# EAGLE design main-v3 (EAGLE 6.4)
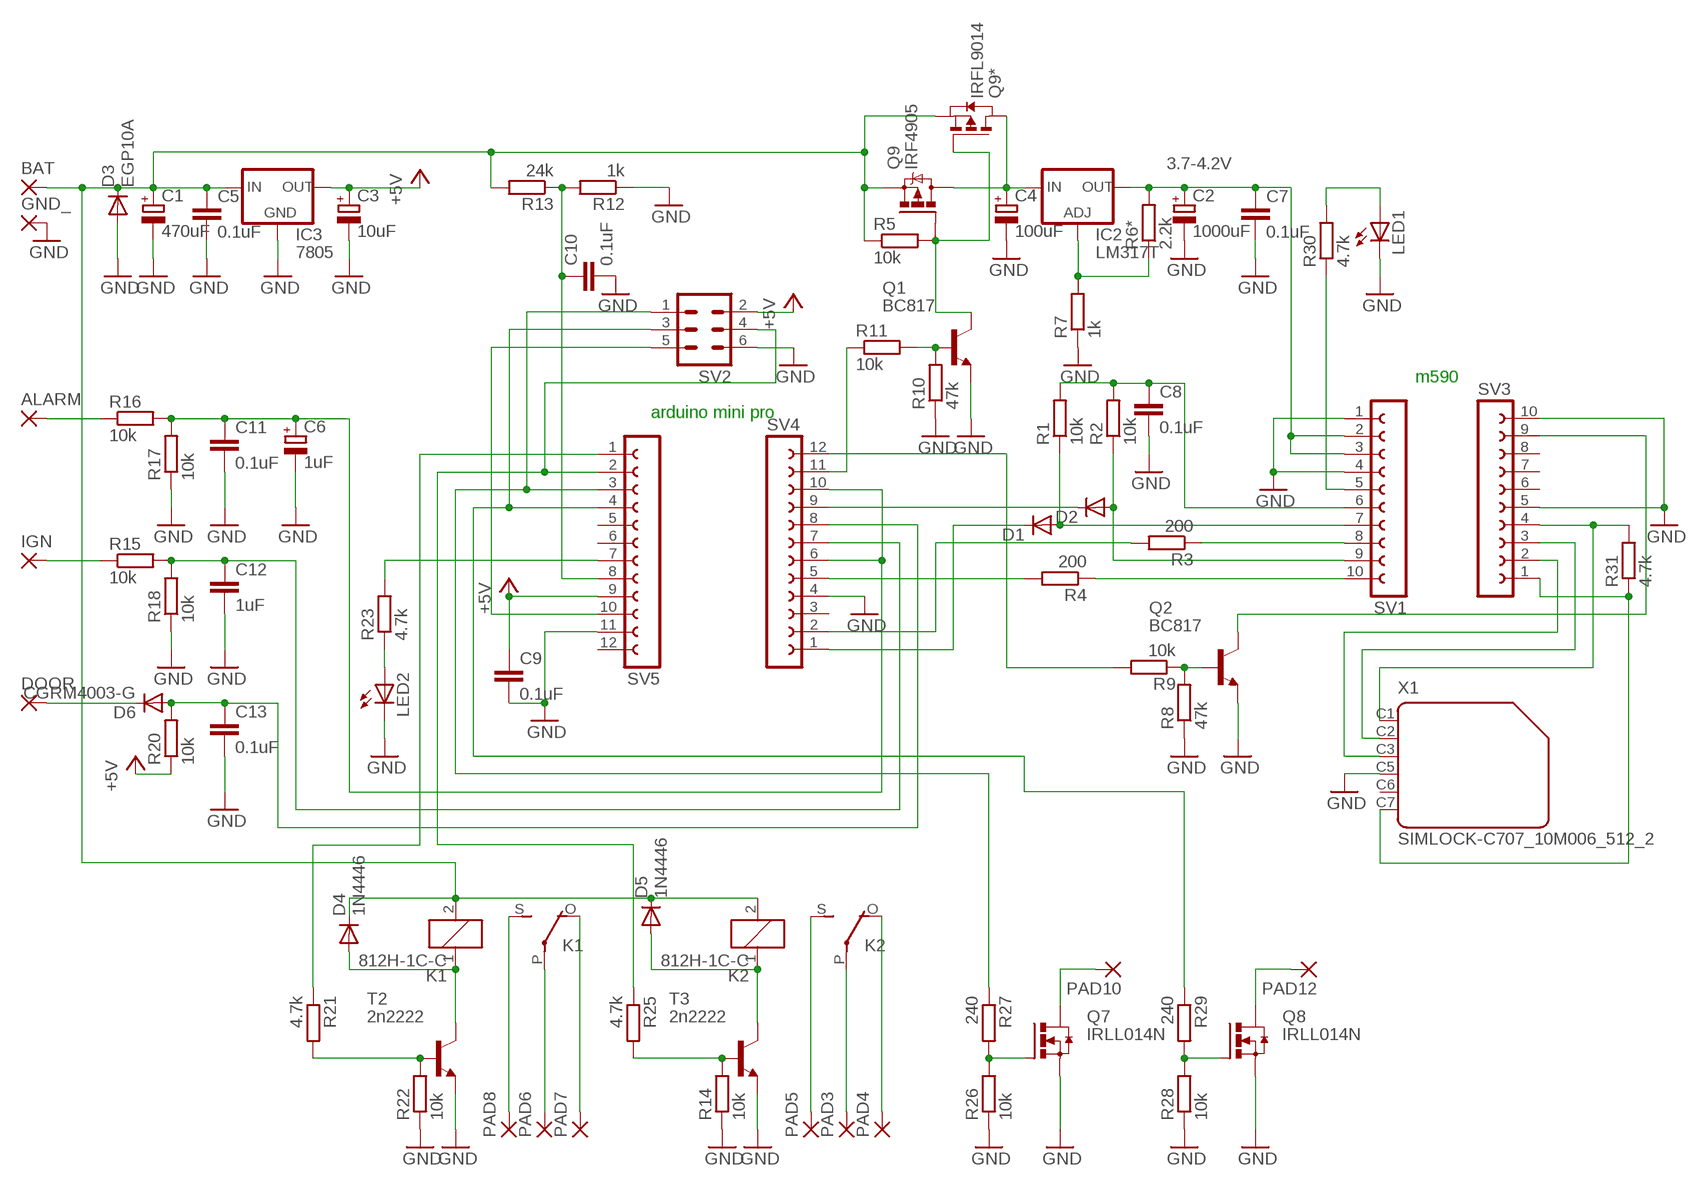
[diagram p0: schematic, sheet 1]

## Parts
ALARM  3,17/1,1  [3,17/1,1]
BAT  3,17/1,1  [3,17/1,1]
C1  470uF  CPOL-EUE5-10.5  [E5-10,5]
C2  1000uF  CPOL-EUE2.5-7  [E2,5-7]
C3  10uF  CPOL-EUE2.5-7  [E2,5-7]
C4  100uF  CPOL-EUE2.5-7  [E2,5-7]
C5  0.1uF  C-EUC1206  [C1206]
C6  1uF  CPOL-EUE2.5-7  [E2,5-7]
C7  0.1uF  C-EUC1206  [C1206]
C8  0.1uF  C-EUC1206  [C1206]
C9  0.1uF  C-EUC1206  [C1206]
C10  0.1uF  C-EUC1206  [C1206]
C11  0.1uF  C-EUC1206  [C1206]
C12  1uF  C-EUC1206  [C1206]
C13  0.1uF  C-EUC1206  [C1206]
D1  BAS15  [DO34-7]
D2  BAS15  [DO34-7]
D3  EGP10A  [DO41-10]
D4  1N4446  [DO35-10]
D5  1N4446  [DO35-10]
D6  CGRM4003-G  [SOD-123_MINI-SMA]
DOOR  3,17/1,1  [3,17/1,1]
GND_  3,17/1,1  [3,17/1,1]
IC2  LM317T  LM317TL  [317TL]
IC3  7805  78XXL  [78XXL]
IGN  3,17/1,1  [3,17/1,1]
K1  812H-1C-C  G5LE  [G5LE]
K2  812H-1C-C  G5LE  [G5LE]
LED1  LED3MM  [LED3MM]
LED2  LED3MM  [LED3MM]
PAD3  3,17/1,1  [3,17/1,1]
PAD4  3,17/1,1  [3,17/1,1]
PAD5  3,17/1,1  [3,17/1,1]
PAD6  3,17/1,1  [3,17/1,1]
PAD7  3,17/1,1  [3,17/1,1]
PAD8  3,17/1,1  [3,17/1,1]
PAD10  3,17/1,1  [3,17/1,1]
PAD12  3,17/1,1  [3,17/1,1]
Q1  BC817  BC817-16LT1SMD  [SOT23-BEC]
Q2  BC817  BC817-16LT1SMD  [SOT23-BEC]
Q7  IRLL014N  N-HEXFET_SOT323-IRLL014N  [SOT223]
Q8  IRLL014N  N-HEXFET_SOT323-IRLL014N  [SOT223]
Q9  IRF4905  [TO220BH]
Q9*  IRFL9014  PMOSSOT223  [SOT223]
R1  10k  R-EU_M1206  [M1206]
R2  10k  R-EU_M1206  [M1206]
R3  200  R-EU_M1206  [M1206]
R4  200  R-EU_0207/10  [0207/10]
R5  10k  R-EU_M1206  [M1206]
R6*  2.2k  R-EU_M1206  [M1206]
R7  1k  R-EU_M1206  [M1206]
R8  47k  R-EU_M1206  [M1206]
R9  10k  R-EU_M1206  [M1206]
R10  47k  R-EU_M1206  [M1206]
R11  10k  R-EU_0207/10  [0207/10]
R12  1k  R-EU_M1206  [M1206]
R13  24k  R-EU_M1206  [M1206]
R14  10k  R-EU_M1206  [M1206]
R15  10k  R-EU_M1206  [M1206]
R16  10k  R-EU_M1206  [M1206]
R17  10k  R-EU_0207/10  [0207/10]
R18  10k  R-EU_0207/10  [0207/10]
R20  10k  R-EU_0207/10  [0207/10]
R21  4.7k  R-EU_M1206  [M1206]
R22  10k  R-EU_M1206  [M1206]
R23  4.7k  R-EU_M1206  [M1206]
R25  4.7k  R-EU_M1206  [M1206]
R26  10k  R-EU_M1206  [M1206]
R27  240  R-EU_M1206  [M1206]
R28  10k  R-EU_M1206  [M1206]
R29  240  R-EU_M1206  [M1206]
R30  4.7k  R-EU_M1206  [M1206]
R31  4.7k  R-EU_M1206  [M1206]
SV1  FE10-1  [FE10]
SV2  MA03-2  [MA03-2]
SV3  FE10-1  [FE10]
SV4  FE12-1  [FE12]
SV5  FE12-1  [FE12]
T2  2n2222  MPS2222A-NPN-TO92-CBE  [TO92-CBE]
T3  2n2222  MPS2222A-NPN-TO92-CBE  [TO92-CBE]
X1  SIMLOCK-C707_10M006_512_2  [C707_10M006_512_2]

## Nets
+5V: C3.+ C9.1 IC3.OUT R20.1 SV2.2 SV5.9
GND: C1.- C2.- C3.- C4.- C5.2 C6.- C7.2 C8.2 C9.2 C10.2 C11.2 C12.2 C13.2 D3.A GND_.1(P) IC3.GND LED1.K(C) LED2.K(C) Q1.E Q2.E Q7.3(S) Q8.3(S) R7.1 R8.1 R10.1 R12.1 R14.1 R17.1 R18.1 R22.1 R26.1 R28.1 SV1.1 SV1.4 SV2.6 SV3.5 SV3.10 SV4.4 SV5.11 T2.E T3.E X1.C5
N$2: D2.A R2.1 SV1.9
N$3: D1.A R1.1 SV1.7
N$4: R3.1 SV1.8
N$5: R4.1 SV1.10
N$6: IC2.1(ADJ) R6*.1 R7.2
N$7: Q1.C Q9*.1(G) Q9.G R5.2
N$8: C4.+ IC2.3(IN) Q9*.2(D) Q9*.4(D) Q9.D
N$9: C12.1 R15.2 R18.2 SV4.7
N$10: Q2.C SV3.9
N$11: R3.2 SV4.2
N$12: R4.2 SV4.5
N$13: D1.C SV4.1
N$14: Q1.B R10.2 R11.2
N$15: Q2.B R8.2 R9.1
N$16: R9.2 SV4.12
N$17: D2.C SV4.9
N$18: R11.1 SV4.11
N$19: C10.1 R12.2 R13.1 SV5.8
N$20: LED1.A R30.2
N$21: BAT.1(P) C1.+ C5.1 D3.C D4.C D5.C IC3.IN K1.2 K2.2 Q9*.3(S) Q9.S R5.1 R13.2
N$22: R30.1 SV1.5
N$23: K1.S(2:S) PAD8.1(P)
N$24: K1.O(2:O) PAD7.1(P)
N$25: K1.P(2:P) PAD6.1(P)
N$26: LED2.A R23.1
N$27: ALARM.1(P) R16.1
N$28: R29.1 SV2.3 SV5.4
N$29: C6.+ C11.1 R16.2 R17.2 SV4.6 SV4.10
N$30: IGN.1(P) R15.1
N$31: D6.C DOOR.1(P)
N$32: C13.1 D6.A R20.2 SV4.8
N$33: SV2.5 SV5.10
N$34: R21.2 R22.2 T2.B
N$35: D5.A K2.1 T3.C
N$36: R14.2 R25.2 T3.B
N$37: R23.2 SV5.7
N$38: R25.1 SV2.4 SV5.2
N$39: K2.S(2:S) PAD5.1(P)
N$40: K2.O(2:O) PAD4.1(P)
N$41: K2.P(2:P) PAD3.1(P)
N$42: R31.1 SV3.1 X1.C7
N$43: R21.1 SV5.1
N$45: R31.2 SV3.4 X1.C1
N$46: Q7.1(G) R26.2 R27.2
N$47: Q8.1(G) R28.2 R29.2
N$48: PAD10.1(P) Q7.4(D)
N$49: PAD12.1(P) Q8.4(D)
N$50: R27.1 SV2.1 SV5.3
N$51: C2.+ C7.1 IC2.2(OUT) R6*.2 SV1.2 SV1.3
N$52: C8.1 R1.2 R2.2 SV1.6
N$53: SV3.3 X1.C2
N$54: SV3.2 X1.C3
N$62: D4.A K1.1 T2.C
Unconnected: SV3.6 SV3.7 SV3.8 SV4.3 SV5.5 SV5.6 SV5.12 X1.C6

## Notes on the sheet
- 3.7-4.2V
- m590
- arduino mini pro

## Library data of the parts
ALARM BAT DOOR GND_ IGN PAD3-PAD8 PAD10 PAD12 = wirepad:3,17/1,1: THROUGH-HOLE PAD
C1-C4 C6 = rcl:CPOL-EU: POLARIZED CAPACITOR, European symbol
C5 C7-C13 = rcl:C-EU: CAPACITOR, European symbol
D1 D2 = diode:BAS15: DIODE
D3 = diode:EGP10A: DIODE
D4 D5 = diode:1N4446: DIODE
D6 = diode:CGRM400*-G: Molded plasitc,JEDEC SOD-123/Mini SMA
IC2 = v-reg-3:LM317TL: VOLTAGE REGULATOR
IC3 = v-reg:78XXL: VOLTAGE REGULATOR
K1 K2 = relay:G5LE: RELAY 1 x switch, 10 A/120 V AC, 8 A/30 V DC, Omron; OC_FARNELL: unknown; OC_NEWARK: unknown
LED1 LED2 = led:LED: LED
Q1 Q2 = transistor-npn:BC817*: NPN Transistor
Q7 Q8 = transistor-power:N-HEXFET_?-*: HEXFET® Power MOSFET
Q9 = transistor-power:IRF4905: P-Channel HEXFET® Power MOSFET RDS(on)= 0.02 Ohm, ID = -74A Source: http://www.irf.com/product-info/datasheets/data/irf4905pbf.pdf
Q9* = zetex:PMOSSOT223: MOS FET; OC_FARNELL: unknown; OC_NEWARK: unknown
R1-R5 R6* R7-R18 R20-R23 R25-R31 = rcl:R-EU_: RESISTOR, European symbol
SV1 SV3 = con-lsta:FE10-1: FEMALE HEADER; OC_FARNELL: unknown; OC_NEWARK: unknown
SV2 = con-lstb:MA03-2: PIN HEADER; OC_FARNELL: unknown; OC_NEWARK: unknown
SV4 SV5 = con-lsta:FE12-1: FEMALE HEADER; OC_FARNELL: unknown; OC_NEWARK: unknown
T2 T3 = transistor:*-NPN-: NPN Transistror BF959 corrected 2008.03.06
X1 = con-amphenol:SIMLOCK-C707_10M006_512_2: C707A SIMLOCK® 2.5 mm with wide solder tails Source: Data sheet; OC_FARNELL: unknown; OC_NEWARK: unknown

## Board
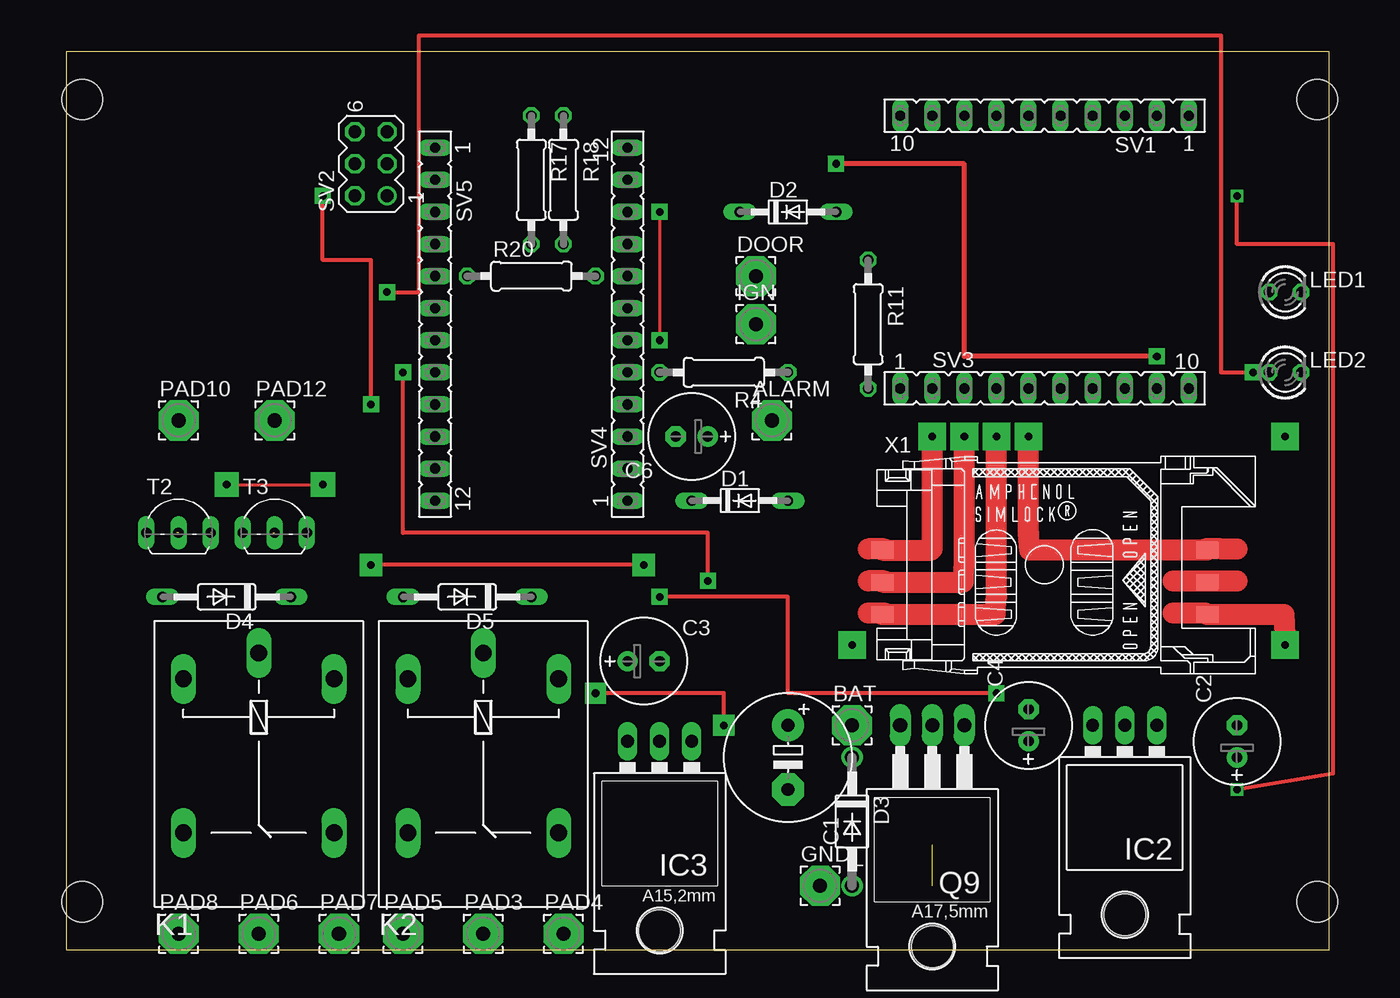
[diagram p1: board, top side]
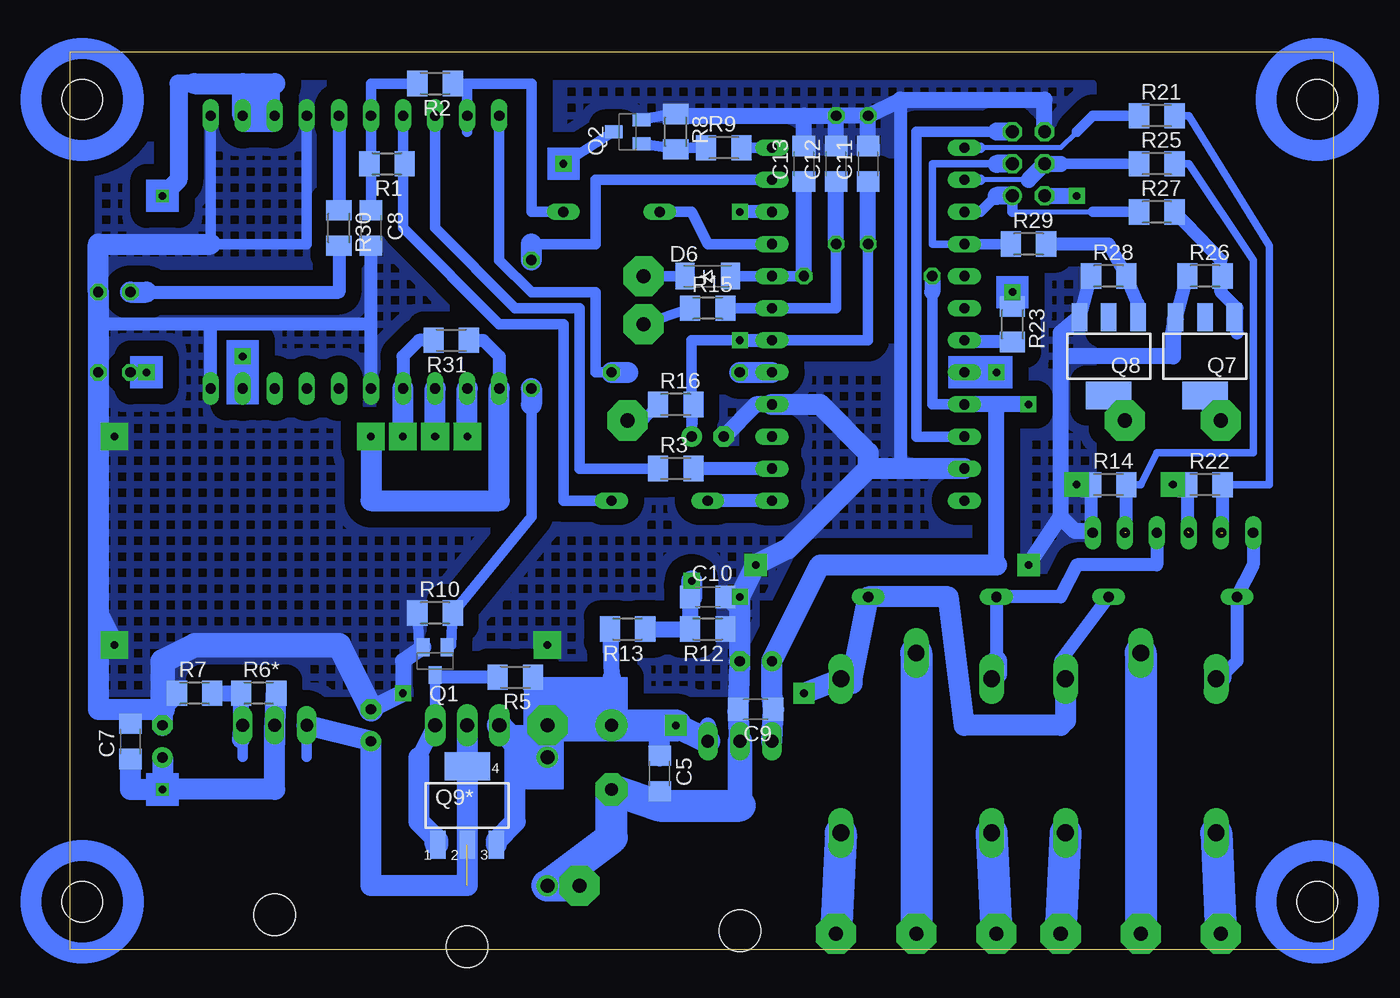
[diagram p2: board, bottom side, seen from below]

Size 100 x 71.11 mm. Coordinates in mm from the lower left corner, seen from the top.
Outline: 0,0 100,0 100,71.11 0,71.11 0,0
Copper layers (1*16): Top 0.035mm / dielectric 1.5mm / Bottom 0.035mm
Design rules "default": minimum track width 10mil, minimum drill 24mil, track to track 8mil, track to pad 8mil, pad to pad 8mil, via to via 8mil, smd to smd 8mil, copper to edge 40mil, drill to drill 8mil, minimum pad ring 10mil, minimum via ring 8mil, stop-mask expansion 4mil, vias tented up to drill 0mil, thermal gap 10mil
Holes 3.2 mm at 1.27,67.31 99.06,67.31 1.27,3.81 99.06,3.81

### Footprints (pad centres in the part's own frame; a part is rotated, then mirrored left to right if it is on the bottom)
3,17/1,1 = drill 1.118 pad 3.175 octagon: 1 0,0
E5-10,5 = drill 1.016 pad 2.54: + -2.54,0 | drill 1.016 pad 2.54 octagon: - 2.54,0
E2,5-7 = drill 0.813 pad 1.6: + -1.27,0 | drill 0.813 pad 1.6 octagon: - 1.27,0
C1206 = smd 1.6 x 1.8: 1 -1.4,0; 2 1.4,0
DO34-7 = drill 0.813 long: A 3.81,0; C -3.81,0
DO41-10 = drill 1.118: A 5.08,0; C -5.08,0
DO35-10 = drill 0.813 long: A 5.08,0; C -5.08,0
SOD-123_MINI-SMA = smd 1.5 x 2.1: A 1.8,0; C -1.8,0
317TL = drill 1.016 long: 1 -2.54,-3.81; 2 0,-3.81; 3 2.54,-3.81 | hole 3.302: 0,11.176
78XXL = drill 1.016 long: GND 0,-3.81; IN -2.54,-3.81; OUT 2.54,-3.81 | hole 3.302: 0,11.176
G5LE = drill 1.321 long: 1 -7.493,-5.969; 2 -7.493,5.969; O 4.699,5.969; P -9.525,0; S 4.699,-5.969
LED3MM = drill 0.813 octagon: A -1.27,0; K 1.27,0
SOT23-BEC = smd 1 x 1.4: B -0.95,-1.1; C 0,1.1; E 0.95,-1.1
SOT223 = smd 1.219 x 2.235: 1 -2.311,-3.099; 2 0,-3.099; 3 2.311,-3.099 | smd 3.6 x 2.2: 4 0,3.099
TO220BH = drill 1.118 long: D 0,-6.35; G -2.54,-6.35; S 2.54,-6.35 | hole 3.302: 0,11.176
M1206 = smd 1.6 x 2: 1 -1.4,0; 2 1.4,0
0207/10 = drill 0.813 octagon: 1 -5.08,0; 2 5.08,0
FE10 = drill 0.813 long: 1 -11.43,0; 2 -8.89,0; 3 -6.35,0; 4 -3.81,0; 5 -1.27,0; 6 1.27,0; 7 3.81,0; 8 6.35,0; 9 8.89,0; 10 11.43,0
MA03-2 = drill 1.016: 1 -2.54,-1.27 | drill 1.016 octagon: 2 -2.54,1.27; 3 0,-1.27; 4 0,1.27; 5 2.54,-1.27; 6 2.54,1.27
FE12 = drill 0.813 long: 1 -13.97,0; 2 -11.43,0; 3 -8.89,0; 4 -6.35,0; 5 -3.81,0; 6 -1.27,0; 7 1.27,0; 8 3.81,0; 9 6.35,0; 10 8.89,0; 11 11.43,0; 12 13.97,0
TO92-CBE = drill 0.813 long: B 0,0; C -2.54,0; E 2.54,0
C707_10M006_512_2 = smd 1.7 x 1.3: C1 -12.85,-3.915; C2 -12.85,-1.375; C3 -12.85,1.165; C5 12.85,-3.915; C6 12.85,-1.375; C7 12.85,1.165

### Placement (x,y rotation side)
ALARM  55.88,41.91 0 top
BAT  62.23,17.78 0 top
C1  57.15,15.24 270 top
C2  92.71,16.51 90 top
C3  45.72,22.86 0 top
C4  76.2,17.78 90 top
C5  53.34,13.97 270 bottom
C6  49.53,40.64 180 top
C7  95.25,16.51 90 bottom
C8  76.2,57.15 270 bottom
C9  45.72,19.05 180 bottom
C10  49.53,27.94 0 bottom
C11  36.83,62.23 90 bottom
C12  39.37,62.23 90 bottom
C13  41.91,62.23 90 bottom
D1  53.34,35.56 0 top
D2  57.15,58.42 0 top
D3  62.23,10.16 270 top
D4  12.7,27.94 180 top
D5  31.75,27.94 180 top
D6  49.53,53.34 0 bottom
DOOR  54.61,53.34 0 top
GND_  59.69,5.08 0 top
IC2  83.82,13.97 180 top
IC3  46.99,12.7 180 top
IGN  54.61,49.53 0 top
K1  15.24,13.97 270 top
K2  33.02,13.97 270 top
LED1  96.52,52.07 0 top
LED2  96.52,45.72 0 top
PAD3  33.02,1.27 0 top
PAD4  39.37,1.27 0 top
PAD5  26.67,1.27 0 top
PAD6  15.24,1.27 0 top
PAD7  21.59,1.27 0 top
PAD8  8.89,1.27 0 top
PAD10  8.89,41.91 0 top
PAD12  16.51,41.91 0 top
Q1  71.12,22.86 180 bottom
Q2  55.88,64.77 90 bottom
Q7  10.16,46.99 180 bottom
Q8  17.78,46.99 180 bottom
Q9  68.58,11.43 180 top
Q9*  68.58,11.43 0 bottom
R1  74.93,62.23 180 bottom
R2  71.12,68.58 180 bottom
R3  52.07,38.1 0 bottom
R4  52.07,45.72 180 top
R5  64.77,21.59 180 bottom
R6*  85.09,20.32 0 bottom
R7  90.17,20.32 0 bottom
R8  52.07,64.77 270 bottom
R9  48.26,63.5 0 bottom
R10  71.12,26.67 0 bottom
R11  63.5,49.53 270 top
R12  49.53,25.4 180 bottom
R13  55.88,25.4 180 bottom
R14  17.78,36.83 0 bottom
R15  49.53,50.8 0 bottom
R16  52.07,43.18 0 bottom
R17  36.83,60.96 270 top
R18  39.37,60.96 270 top
R20  36.83,53.34 0 top
R21  13.97,66.04 0 bottom
R22  10.16,36.83 0 bottom
R23  25.4,49.53 270 bottom
R25  13.97,62.23 0 bottom
R26  10.16,53.34 0 bottom
R27  13.97,58.42 0 bottom
R28  17.78,53.34 0 bottom
R29  24.13,55.88 0 bottom
R30  78.74,57.15 270 bottom
R31  69.85,48.26 180 bottom
SV1  77.47,66.04 180 top
SV2  24.13,62.23 90 top
SV3  77.47,44.45 0 top
SV4  44.45,49.53 90 top
SV5  29.21,49.53 270 top
T2  8.89,33.02 0 top
T3  16.51,33.02 0 top
X1  77.47,30.48 0 top

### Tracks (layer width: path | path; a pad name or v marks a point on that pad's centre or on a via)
+5V  (via drill 0.6 pad 1.27)
  Top 0.305: v24.13,43.18 24.13,54.61 20.32,54.61 v20.32,59.69
  Bottom 0.813: 31.75,52.07 31.75,43.18 SV5.9
  Bottom 1.27: 26.67,30.48 26.67,43.18 | 26.67,43.18 SV5.9 | SV2.2 v20.32,59.69 | v24.13,43.18 26.67,43.18 | R20.1 31.75,52.07
  Bottom 1.676: 26.67,30.48 40.64,30.48 C3.+ 44.45,20.32 C9.1 IC3.OUT
GND  (via drill 0.6 pad 1.27, 0.6 pad 1.78, 0.6 pad 1.93, 0.6 pad 2.18)  (1 unrouted)
  Top 0.254: v12.7,36.83 v20.32,36.83
  Top 0.305: v73.66,20.32 57.15,20.32 57.15,27.94 v46.99,27.94 | v45.72,30.48 v24.13,30.48
  Top 1.676: X1.C5 96.42,26.56 v96.52,24.13
  Bottom 0.813: 52.07,66.04 53.19,66.04 Q2.E | Q1.E 72.39,24.13 R10.1 | SV1.4 81.28,55.88 88.9,55.88 SV1.1
  Bottom 1.016: R26.1 12.47,49.89 12.7,49.89 12.7,48.26 | Q8.3 20.09,49.89 R28.1 | SV3.5 76.2,49.53 | 76.2,49.53 88.9,49.53 | 88.9,49.53 97.79,49.53 | SV3.10 88.9,49.53 | 76.2,49.53 C8.2 | 19.05,36.83 R14.1 19.18,33.15 T3.E | R22.1 11.56,33.15 | 34.29,67.31 34.29,38.1 | R12.1 46.99,25.4 | C10.2 48.13,27.81 46.99,26.67
  Bottom 1.27: R17.1 R18.1 | R8.1 52.07,66.04 41.91,66.04 | C12.2 R18.1 | C11.2 R17.1 | SV2.6 22.86,67.31 34.29,67.31 R17.1 | SV4.4 45.72,43.18 C6.- | Q1.E 73.66,22.86 v73.66,20.32 | Q7.3 12.7,48.82 12.7,48.26 12.7,46.99 21.59,46.99 | 21.59,46.99 21.59,34.29 | v24.13,30.48 21.59,34.29 | Q8.3 21.59,48.82 21.59,46.99 | C5.2 53.34,11.43 | R22.1 v12.7,36.83 | v20.32,36.83 R14.1 | 19.18,33.15 20.45,33.15 21.59,34.29 | 41.91,66.04 R18.1 | C13.2 41.91,66.04
  Bottom 1.422: v73.66,20.32 C4.- | 92.71,19.05 R7.1 | C7.2 95.25,19.05
  Bottom 1.676: 88.9,55.88 97.79,55.88 LED1.K 97.79,49.53 97.79,40.64 | 97.79,40.64 97.79,26.67 | 97.79,26.67 97.79,19.05 95.25,19.05 92.71,19.05 C2.- | v96.52,24.13 97.79,26.67 | IC3.GND C9.2 47.03,22.82 C3.- 46.99,25.4 46.99,26.67 v46.99,27.94 v45.72,30.48 43.18,31.75 36.83,38.1 | SV5.11 34.29,38.1 36.83,38.1 | SV4.4 40.64,43.18 36.83,39.37 36.83,38.1 | v96.52,40.64 97.79,40.64
  Bottom 1.93: C4.- 78.74,24.13 90.17,24.13 92.71,22.86 92.71,19.05 | IC3.GND 46.99,11.43
  Bottom 2.54: GND_.1 D3.A 57.15,8.89 C1.- 53.34,11.43 46.99,11.43
  other vias: 62.23,24.13
  pour Bottom (isolate 1.27, no thermals, hatched): 19.05,68.58 97.79,68.58 97.79,20.32 45.72,20.32 45.72,27.94 19.05,27.94
N$1
  Top 1.676: 64.77,31.75 63.5,31.75
N$2
  Bottom 0.813: 68.58,64.77 SV1.9 68.58,68.58 | D2.A 63.5,58.42 63.5,68.58 68.58,68.58 | R2.1 68.58,68.58
N$3
  Bottom 0.813: D1.A 60.96,35.56 60.96,49.53 66.04,49.53 73.66,57.15 73.66,62.23 R1.1 73.66,62.36 SV1.7
N$4
  Bottom 0.813: SV1.8 71.12,57.15 64.77,50.8 59.69,50.8 59.69,38.1 R3.1
N$5
  Bottom 0.813: SV1.10 66.04,54.61 63.5,52.07 58.42,52.07 58.42,45.72 R4.1
  Bottom 1.676: R4.1 55.88,45.72
N$6
  Bottom 0.813: 86.36,15.3 IC2.1
  Bottom 1.27: 86.49,16.64 R6*.1 R7.2
  Bottom 1.422: 86.49,16.64 IC2.1
N$7
  Bottom 0.813: Q1.C 71.12,21.59 Q9.G
  Bottom 1.016: R5.2 71.12,21.59
  Bottom 1.27: Q9*.1 71.12,8.33 | 72.39,15.24 Q9.G
  Bottom 1.676: Q9*.1 70.89,8.66 71.12,8.89 | 71.12,8.33 71.12,8.89 | 71.12,8.89 72.39,10.16 72.39,15.24
N$8  (1 unrouted)
  Bottom 0.813: 81.28,15.3 IC2.3
  Bottom 1.676: IC2.3 C4.+ 76.2,5.08 68.58,5.08 Q9*.4 Q9.D
N$9
  Bottom 0.813: R18.2 39.37,50.8 SV4.7 R15.2
  Bottom 1.27: R18.2 C12.1
N$10  (via drill 0.6 pad 1.27)
  Top 0.406: v86.36,46.99 71.12,46.99 71.12,62.23 v60.96,62.23
  Bottom 0.813: Q2.C v60.96,62.23
  Bottom 1.27: SV3.9 v86.36,46.99
N$11
  Bottom 1.016: 46.99,38.1 SV4.2 R3.2
N$12
  Bottom 1.676: R4.2 SV4.5
N$13
  Bottom 1.016: SV4.1 D1.C
N$14
  Bottom 0.813: 63.5,43.18 63.5,34.29 R10.2 69.85,24.13 Q1.B
  Bottom 1.676: R11.2 63.5,43.18
N$15
  Bottom 0.813: R9.1 50.93,63.5 R8.2 51.79,63.37 Q2.B
N$16
  Bottom 0.813: R9.2 SV4.12
N$17
  Bottom 0.813: SV4.9 49.53,55.88 50.8,58.42 D2.C
N$18
  Bottom 0.813: 63.5,55.88 58.42,55.88 58.42,60.96 SV4.11
  Bottom 1.676: R11.1 63.5,55.88
N$19  (via drill 0.6 pad 1.27)
  Top 0.305: v50.8,29.21 50.8,33.02 26.67,33.02 v26.67,45.72
  Bottom 0.813: C10.1 50.8,27.94
  Bottom 1.016: v26.67,45.72 SV5.8
  Bottom 1.27: R13.1 R12.2 C10.1
  Bottom 1.676: v50.8,29.21 50.8,27.94
N$20
  Bottom 1.016: R30.2 78.74,52.07 93.98,52.07
  Bottom 1.676: LED1.A 93.98,52.07
N$21  (via drill 0.6 pad 1.68)
  Top 0.305: v52.07,17.78 52.07,20.32 v41.91,20.32
  Bottom 1.016: D4.C 21.59,22.86 21.59,21.84 K1.2
  Bottom 1.27: 49.53,17.78 IC3.IN | R13.2 57.15,21.59
  Bottom 1.422: R5.1 63.5,16.51 | 57.15,21.59 C1.+
  Bottom 1.676: Q9.S 64.77,16.51 | 64.77,16.51 63.5,16.51 BAT.1 | Q9*.3 66.27,8.66 64.77,10.16 64.77,16.51 | K1.2 21.21,18.16 21.59,17.78 29.21,17.78 30.48,27.94 D5.C 38.1,21.59 38.1,21.08 K2.2 v41.91,20.32 | C5.1 53.34,17.78
  Bottom 1.93: Q9.S 64.77,16.38 | v52.07,17.78 IC3.IN
  Bottom 2.54: D3.C BAT.1 C1.+ 53.34,17.78 v52.07,17.78
N$22
  Bottom 1.016: SV1.5 R30.1
N$23
  Bottom 2.54: K1.S PAD8.1
N$24
  Bottom 2.54: K1.O PAD7.1
N$25
  Bottom 2.54: K1.P PAD6.1
N$26  (via drill 0.6 pad 1.27)
  Top 0.305: v25.4,52.07 27.94,52.07 27.94,72.39 91.44,72.39 91.44,45.72 v93.98,45.72
  Bottom 1.27: R23.1 v25.4,52.07 | v93.98,45.72 LED2.A
N$27
  Bottom 0.813: ALARM.1 54.61,41.91 R16.1
N$28
  Bottom 0.61: SV5.4 31.75,55.88 31.75,62.23 26.67,62.23
  Bottom 0.813: R29.1 SV5.4
  Bottom 1.422: SV2.3 26.67,62.23
N$29  (via drill 0.6 pad 1.27)
  Top 0.254: v46.99,58.42 v46.99,48.26
  Bottom 0.813: SV4.6 36.83,48.26 R17.2 | v46.99,48.26 50.8,48.26 C6.+ R16.2
  Bottom 1.016: SV4.10 v46.99,58.42 | v46.99,48.26 SV4.6
  Bottom 1.27: R17.2 C11.1
N$30
  Bottom 0.813: R15.1 IGN.1
N$31
  Bottom 0.813: DOOR.1 D6.C
N$32
  Bottom 0.813: R20.2 SV4.8 D6.A
  Bottom 1.27: R20.2 C13.1
N$33
  Bottom 0.813: SV5.10 33.02,40.64 33.02,64.77 26.67,64.77
  Bottom 1.422: SV2.5 26.67,64.77
N$34  (1 unrouted)
  Bottom 0.61: R21.2 11.43,66.04 5.08,55.75 5.08,36.83 R22.2
  Bottom 1.016: 8.76,33.02 R22.2
N$35
  Bottom 1.016: 26.67,22.86 D5.A 21.59,27.94 20.32,30.48 13.97,30.48 T3.C
  Bottom 1.676: 26.67,22.86 26.67,21.84 K2.1
N$36  (1 unrouted)
  Bottom 0.61: R25.2 11.43,62.23 6.35,54.61 6.35,39.37 13.97,39.37 15.24,36.83 R14.2
  Bottom 1.016: 16.38,33.02 R14.2
N$37
  Bottom 1.016: 25.4,48.26 R23.2 29.08,48.13 SV5.7
N$38
  Bottom 0.406: 24.13,60.96 27.94,60.96
  Bottom 0.813: SV5.2 27.94,60.96 | R25.1 21.59,62.23
  Bottom 1.27: 21.59,62.23 SV2.4 24.13,60.96
N$39
  Bottom 2.54: K2.S PAD5.1
N$40
  Bottom 2.54: K2.O PAD4.1
N$41
  Bottom 2.54: K2.P PAD3.1
N$42  (via drill 0.6 pad 2.18)
  Top 1.676: X1.C7 76.31,31.64 76.2,33.02 v76.2,40.64
  Bottom 1.016: R31.1 67.31,48.26 66.04,46.99 SV3.1
  Bottom 1.676: v76.2,40.64 76.2,35.56 66.04,35.56 SV3.1
N$43
  Bottom 0.406: 27.94,63.5 21.59,63.5 20.32,64.77
  Bottom 0.813: SV5.1 27.94,63.5 | 15.24,66.04 R21.1 19.05,66.04 20.32,64.77
N$45  (via drill 0.6 pad 2.18)
  Top 1.676: X1.C1 73.56,26.56 73.66,27.94 v73.66,40.64
  Bottom 1.016: R31.2 72.39,48.26 73.66,46.99 SV3.4
  Bottom 1.676: v73.66,40.64 SV3.4
N$46
  Bottom 1.016: 8.89,52.07 8.89,54.61 R27.2 | Q7.1 7.62,48.82 7.62,50.8 8.89,52.07 | 8.89,52.07 R26.2
N$47
  Bottom 1.016: Q8.1 15.47,51.16 R28.2 17.78,55.88 R29.2
N$48
  Bottom 1.676: PAD10.1 Q7.4
N$49
  Bottom 1.016: Q8.4 PAD12.1
N$50
  Bottom 0.406: 25.4,58.42 19.05,58.42
  Bottom 0.813: SV2.1 25.4,58.42 | 26.67,59.69 27.94,58.42 SV5.3 | R27.1 19.05,58.42
  Bottom 1.422: SV2.1 26.67,59.69
N$51  (via drill 0.6)
  Top 0.305: v92.71,12.7 100.33,13.97 100.33,55.88 92.71,55.88 v92.71,59.69
  Bottom 0.813: 83.82,68.58 SV1.3
  Bottom 1.422: 83.82,17.65 R6*.2 | 90.17,68.58 91.44,68.58 91.44,60.96 v92.71,59.69
  Bottom 1.676: R6*.2 83.82,16.38 IC2.2 83.82,12.7 v92.71,12.7 | 90.17,68.58 86.36,68.58 | 86.36,68.58 83.82,68.58 | SV1.2 86.36,68.58 | C7.1 95.25,12.7 v92.71,12.7 | C2.+ v92.71,12.7
N$52
  Bottom 0.813: R2.2 76.2,68.58 SV1.6 76.2,62.23 | 76.2,62.23 C8.1 | R1.2 76.2,62.23
N$53  (via drill 0.6 pad 2.18)
  Top 1.676: X1.C2 71.02,29.1 71.12,30.48 v71.12,40.64
  Bottom 1.676: v71.12,40.64 SV3.3
N$54  (via drill 0.6 pad 2.18)
  Top 1.676: X1.C3 68.47,31.64 68.58,31.75 v68.58,40.64
  Bottom 1.676: v68.58,40.64 SV3.2
N$55
  Top 1.676: 64.77,29.21 63.5,29.21
N$56
  Top 1.676: 64.77,26.67 63.5,26.67
N$57
  Top 1.676: 90.17,26.67 87.63,26.67
N$58
  Top 1.676: 87.63,29.21 92.71,29.21
N$59
  Top 1.676: 90.17,31.75 91.44,31.75 92.71,31.75
N$62
  Bottom 1.016: 9.14,21.59 9.27,21.59 K1.1 9.14,21.59 | T2.C 6.35,30.48 D4.A 7.62,22.86 8.89,21.59 9.14,21.59
  Bottom 1.676: 8.89,21.59 K1.1
(copper drawn outside any net)
  shapes: Bottom area x11, Bottom circle x4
